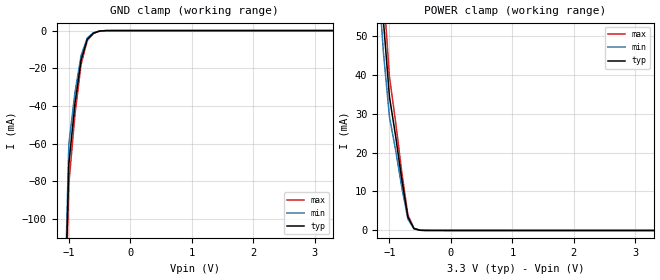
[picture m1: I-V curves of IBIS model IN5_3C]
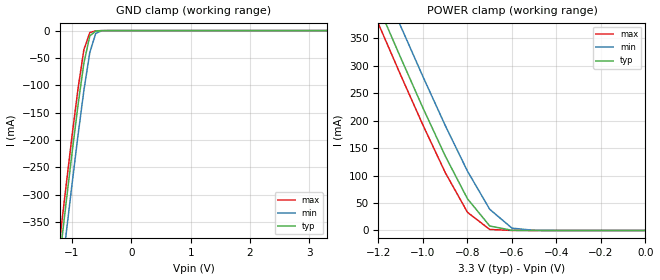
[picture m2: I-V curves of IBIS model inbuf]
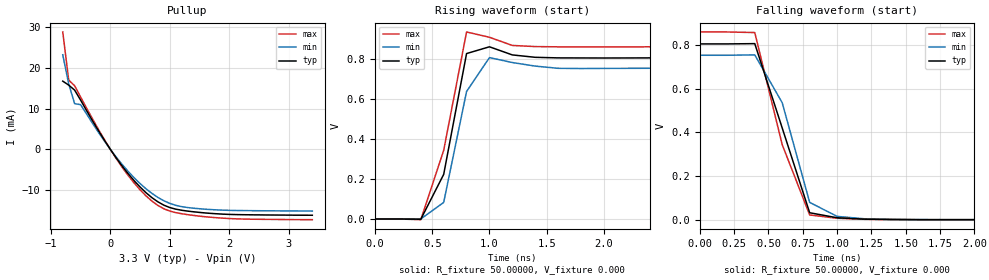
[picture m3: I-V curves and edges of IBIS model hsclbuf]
| IBIS file 5v41068a.ibs created by s2ibis2 version 1.2
| North Carolina State University Electronics Research Laboratory  1995
[IBIS ver]   2.1
[File name]   5v41068a.ibs
[File Rev]   1.1
[Date]   May 3, 2012
|   Corrected non-monotonic warnings. lfp
|[File Rev]   1.0
|[Date]   October 21, 2011   Intial release
[Source]   IDT
[Notes]   1. Temp typ=25C, min=70C, max=0C 2. Ramp rates based on 50 ohm
   load
[Disclaimer] READ THESE TERMS AND CONDITIONS CAREFULLY BEFORE USING THIS
   IBIS MODEL. BY USING THIS IBIS MODEL, YOU ARE ACCEPTING AND
   AGREEING TO THESE TERMS AND CONDITIONS OF USE. Integrated
   Device Technology, Inc. ("IDT") hereby grants the user of this
   IBIS model ("User") a non-exclusive, nontransferable license
   to use this IBIS model under the following terms: The User is
   granted this license only to use the IBIS model for
   demonstration purposes only and is not granted rights to sell,
   copy (except as needed to run the IBIS model), rent, lease or
   sub-license (except for demonstration) the IBIS model in whole
   or in part, or in modified form to anyone. The User may modify
   the IBIS model to suit its specific applications, but rights
   to derivative works and such modifications shall belong to
   IDT. THIS IBIS MODEL IS PROVIDED ON AN AS IS" BASIS AND IDT
   MAKES ABSOLUTELY NO WARRANTY WITH RESPECT TO THE INFORMATION
   CONTAINED HEREIN. IDT DISCLAIMS AND USER WAIVES ALL
   WARRANTIES, EXPRESS AND IMPLIED, INCLUDING WARRANTIES OF
   MERCHANTABILITY AND FITNESS FOR A PARTICULAR PURPOSE. THE
   ENTIRE RISK AS TO QUALITY AND PERFORMANCE IS WITH THE USER
   ACCORDINGLY, IN NO EVENT SHALL IDT BE LIABLE FOR ANY DIRECT OR
   INDIRECT DAMAGES, WHETHER IN CONTRACT OR TORT, INCLUDING ANY
   LOST PROFITS OR OTHER INCIDENTAL, CONSEQUENTIAL, EXEMPLARY, OR
   PUNITIVE DAMAGES ARISING OUT OF THE USE OR APPLICATION OF THE
   IBIS MODEL, WHETHER OR NOT IDT HAD NOTICE OF SUCH DAMAGES. IDT
   reserves the right to make changes without notice to any
   product herein to improve reliability, function, or design.
   IDT does not convey any license under patent rights or any
   other intellectual property rights, including those of third
   parties. IDT is not obligated to provide maintenance or
   support for the licensed IBIS model.
   **************************************** This model is for
   IDT5V41068a IDT Clock ****************************************
[Copyright]   Copyright 2006, Integrated Device Technology, Inc. All rights
   reserved.
|   Component IDT5V41068a
[Component]   IDT5V41068a
[Manufacturer]   Integrated Device Technology Inc.
[Package]
| variable   typ   min   max
R_pkg   81.10000m   62.20000m   100.00000m
L_pkg   6.70000nH   4.90000nH   8.50000nH
C_pkg   0.53000pF   0.21000pF   0.85000pF
[Pin]  signal_name   model_name   R_pin   L_pin   C_pin
1   VDD   POWER
2   IN1   IN5_3C
3   IN1B   IN5_3C
4   PDB   inbuf
5   IN2   IN5_3C
6   IN2B   IN5_3C
7   OE   inbuf
8   GND   GND
9   IREF   NC
10   VDD   POWER
11   VDD   POWER
12   GND   GND
13   GND   GND
14   CLK   hsclbuf
15   CLKB   hsclbuf
16   SEL   inbuf
| in   in   dummy
| oe   oe   dummy
[Diff Pin]  inv_pin  vdiff   tdelay_typ  tdelay_min  tdelay_max
2   3   0.000V   0.000s   0.000s   0.000s
5   6   0.000V   0.000s   0.000s   0.000s
14   15   0.000V   0.000s   0.000s   0.000s
| Models and submodels in the file (3): IN5_3C (Input), inbuf (Input), hsclbuf (Open_source)
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|   Model IN5_3C
[Model]   IN5_3C
Model_type   Input
Vinl =0.00V   | Input logic  "low" DC voltage
Vinh=0.70V   | Input logic  "high" DC voltage
|   typ   min   max
C_comp   5pF   4pF   6pF
[Temperature Range]   25.00000   70.00000   0.000
[Voltage Range]   3.30000V   3.13500V   3.46500V
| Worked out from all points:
|   GND clamp passes 1 mA (typ) near -0.57 V on its own axis
|   POWER clamp passes 1 mA (typ) near -0.62 V on its own axis
[GND_clamp]
|Voltage I (typ)   I (min)   I (max)
-3.3V     -3A        -3A        -3A
-1V       -70.99mA   -60.34mA   -81.64mA
-900mV    -38.73mA   -32.92mA   -44.54mA
-800mV    -15.56mA   -13.23mA   -17.89mA
-700mV    -4.62mA    -3.92mA    -5.31mA
-600mV    -1.36mA    -1.16mA    -1.57mA
-500mV    -260uA     -220uA     -300uA
-400mV    -24.9uA    -21uA      -29uA
3.3V      858nA      729nA      986nA
[POWER_clamp]
|Voltage I (typ)   I (min)   I (max)
-3.3V     3A         3A         3A
-1.2V     81.31mA    69.12mA    93.51mA
-1.1V     54.18mA    46.05mA    62.31mA
-1V       34.31mA    29.17mA    39.46mA
-900mV    24.27mA    20.63mA    27.91mA
-800mV    13.12mA    11.15mA    15.08mA
-700mV    3.44mA     2.924mA    3.956mA
-600mV    472uA      401uA      543uA
-500mV    50.5uA     42.9uA     58.1uA
-400mV    6.01uA     5.1uA      6.91uA
3.3V      -5.79uA    -4.9uA     -6.7uA
|   Model inbuf
[Model]   inbuf
Model_type   Input
Vinl =  0.80000V
Vinh =  2.80000V
C_comp   3.40000pF   2.85000pF   3.95000pF
[Temperature Range]   25.00000   70.00000   0.000
[Voltage Range]   3.30000V   3.13500V   3.46500V
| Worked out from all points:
|   GND clamp passes 1 mA (typ) near -0.60 V on its own axis
|   POWER clamp passes 1 mA (typ) near -0.61 V on its own axis
[GND_clamp]
| voltage   I(typ)   I(min)   I(max)
-3.3V     -2.462A    -2.516A    -2.432A
-1.2V     -408.6mA   -466.1mA   -376.9mA
-1.1V     -315.3mA   -372.7mA   -283.7mA
-1V       -224.2mA   -281.2mA   -193mA
-900mV    -137.1mA   -192.5mA   -107.2mA
-800mV    -59.32mA   -109.4mA   -35.08mA
-700mV    -9.869mA   -39.95mA   -3.587mA
-600mV    -842uA     -5.099mA   -483.1uA
-500mV    -115.1uA   -371.4uA   -82.28uA
3.3V      126.6pA    4.065uA    -5.151uA
[POWER_clamp]
| voltage   I(typ)   I(min)   I(max)
-3.3V     2.461A     2.514A     2.431A
-1.2V     407.3mA    464.7mA    375.7mA
-1.1V     314mA      371.3mA    282.3mA
-1V       222.7mA    279.7mA    191.6mA
-900mV    135.6mA    191mA      105.4mA
-800mV    57.64mA    107.9mA    33.04mA
-700mV    8.171mA    38.53mA    1.847mA
-600mV    258.3uA    4.245mA    53.65uA
-500mV    21.3uA     185.2uA    18uA
0V        126.6pA    323.6pA    125.6pA
|   Model hsclbuf
[Model]   hsclbuf
Model_type   Open_source
Polarity   Non-Inverting
Enable   Active-High
Vmeas =  0.35000V
Rref = 50.00000
Vref =  0.000V
C_comp   3.40000pF   2.85000pF   3.95000pF
[Temperature Range]   25.00000   70.00000   0.000
[Voltage Range]   3.30000V   3.13500V   3.46500V
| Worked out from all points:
|   slope of the pullup table from 0 to 0.495 V, typ, clamps not added: 53.9 ohm
|   rising waveform, R_fixture 50.00000, V_fixture 0.000: 20-80 % time 195ps typ, 163ps min, 215ps max; typ from 0 V to 0.806 V
|   falling waveform, R_fixture 50.00000, V_fixture 0.000: 20-80 % time 249ps typ, 230ps min, 241ps max; typ from 0.806 V to 0 V
[Pullup]
| voltage   I(typ)   I(min)   I(max)
-800mV    16.74mA    23.22mA    28.82mA
-700mV    15.77mA    16.05mA    17mA
-600mV    14.54mA    11.21mA    15.6mA
-500mV    12.09mA    10.96mA    12.86mA
-200mV    4.592mA    4.177mA    4.901mA
100mV     -2.128mA   -1.929mA   -2.281mA
400mV     -7.7mA     -6.984mA   -8.261mA
700mV     -11.88mA   -10.83mA   -12.72mA
1V        -14.31mA   -13.29mA   -15.18mA
1.4V      -15.36mA   -14.48mA   -16.25mA
2.1V      -16.04mA   -15.04mA   -17.08mA
3.4V      -16.21mA   -15.18mA   -17.3mA
[Ramp]
| variable   typ   min   max
dV/dt_r   0.48390/0.14004n   0.45264/0.13312n   0.51678/0.11874n
dV/dt_f   0.48366/0.16100n   0.45247/0.17807n   0.51654/0.15404n
R_load = 50.00000
[Rising Waveform]
R_fixture = 50.00000
V_fixture = 0.000
V_fixture_min = 0.000
V_fixture_max = 0.000
| time   V(typ)   V(min)   V(max)
0s        0V         0V         0V
400ps     -1.245mV   110.3uV    -3.578mV
600ps     223.5mV    82.97mV    344.2mV
800ps     829mV      639.1mV    937.2mV
1ns       862.9mV    808.7mV    910.6mV
1.2ns     822.2mV    784mV      869.7mV
1.4ns     810.2mV    766.1mV    864mV
1.6ns     807.3mV    755mV      862.7mV
10ns      806.5mV    754.4mV    861.3mV
[Falling Waveform]
R_fixture = 50.00000
V_fixture = 0.000
V_fixture_min = 0.000
V_fixture_max = 0.000
| time   V(typ)   V(min)   V(max)
0s        806.1mV    754.1mV    860.9mV
400ps     807.4mV    755.9mV    858.2mV
600ps     420.4mV    536.3mV    343.8mV
800ps     31.73mV    79.3mV     21.64mV
1ns       8.713mV    15.08mV    6.327mV
1.2ns     2.276mV    3.998mV    1.628mV
1.4ns     807.5uV    1.469mV    357.8uV
10ns      -5.905uV   -12.28uV   6.645uV
